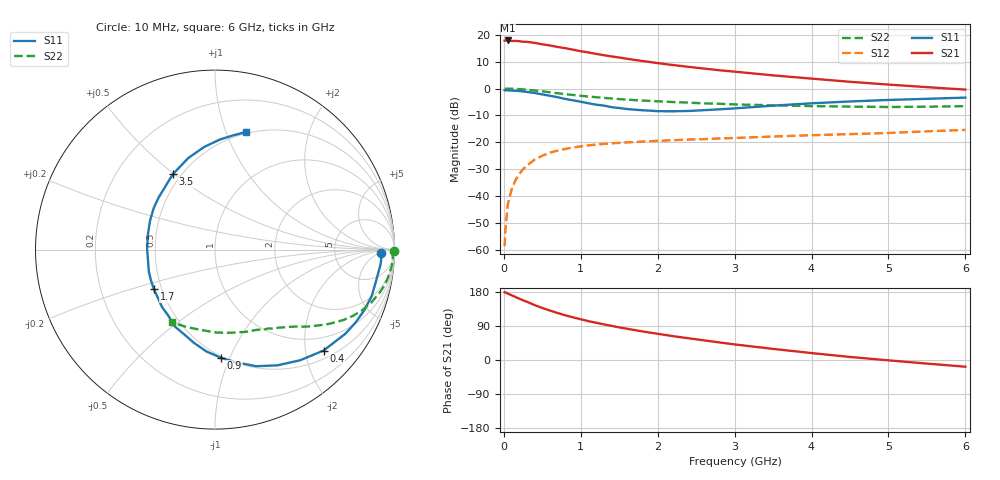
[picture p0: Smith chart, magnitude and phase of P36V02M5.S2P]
! SIEMENS Small Signal Semiconductors
! BFP181
! Si NPN RF Bipolar Junction Transistor in SOT143
! VCE = 6 V  IC = 2.5 mA
! Common Emitter S-Parameters:  March  1996
# GHz  S  MA  R  50
!  f  S11  S21  S12  S22
! GHz  MAG  ANG  MAG  ANG  MAG  ANG  MAG  ANG
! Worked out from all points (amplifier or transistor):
!   36 points, 10 MHz to 6 GHz, reference 50 ohm
!   highest |S21| = 17.8 dB at 50 MHz (marker M1)
!   |S21| within 3 dB of that: start of sweep to 824.2 MHz
!   unconditionally stable (mu >= 1): 2.37 GHz to end of sweep
!   at 250 MHz: K = 0.13, MSG = 23.6 dB, |S12| = -29.9 dB
!   at 1.4 GHz: K = 0.69, MSG = 16.1 dB, |S12| = -20.3 dB
!   at 6 GHz: K = 1.12, MAG = 5.4 dB, |S12| = -15.3 dB
!   S11 on the Smith chart (normalised r, x): 10 MHz: 24, -6; 400 MHz: 0.67, -2.38; 900 MHz: 0.49, -0.93; 1.7 GHz: 0.45, -0.24; 3.5 GHz: 0.45, +0.49; 6 GHz: 0.49, +1.18
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0.01  0.9248 -1.2  7.716 179.0  0.0012 77.8  0.9954 -0.4
0.02  0.9282 -2.3  7.748 178.5  0.0023 89.4  0.9885 -1.0
0.05  0.9263 -5.0  7.765 175.4  0.007 89.0  0.9917 -2.6
0.1  0.9138 -11.4  7.589 170.9  0.0133 81.7  0.9899 -5.1
0.15  0.9105 -16.6  7.629 166.4  0.0198 79.7  0.9816 -7.6
0.2  0.8976 -22.1  7.532 161.9  0.0259 77.0  0.9737 -10.0
0.3  0.8647 -32.8  7.315 153.7  0.0374 70.8  0.9487 -14.6
0.4  0.826 -42.9  7.01 144.9  0.0481 65.2  0.9186 -18.8
0.5  0.7781 -52.4  6.584 137.3  0.0568 59.7  0.8857 -22.5
0.6  0.7324 -61.7  6.277 130.4  0.0648 55.3  0.8521 -25.7
0.8  0.6402 -79.1  5.583 117.9  0.0759 47.9  0.7862 -30.9
0.9  0.6043 -86.7  5.237 112.5  0.081 44.6  0.7578 -33.1
1.1  0.5318 -102.9  4.655 102.5  0.0885 39.7  0.7095 -36.6
1.4  0.4512 -125.1  3.933 90.1  0.0965 34.5  0.6531 -41.1
1.7  0.4056 -147.0  3.388 79.0  0.1017 30.9  0.6096 -44.8
1.9  0.3888 -161.3  3.098 72.3  0.1056 28.5  0.5884 -47.2
2.2  0.3786 179.1  2.719 62.9  0.11 26.8  0.5612 -50.8
2.8  0.4118 146.2  2.179 46.4  0.1188 23.3  0.5216 -58.9
3.5  0.4813 119.2  1.752 29.3  0.129 20.5  0.4889 -69.6
4.5  0.5754 95.9  1.332 8.0  0.1428 16.1  0.4624 -88.9
5.5  0.6442 81.0  1.06 -9.5  0.1609 13.3  0.4595 -109.9
6  0.6781 75.1  0.954 -17.7  0.171 10.8  0.4718 -120.7
